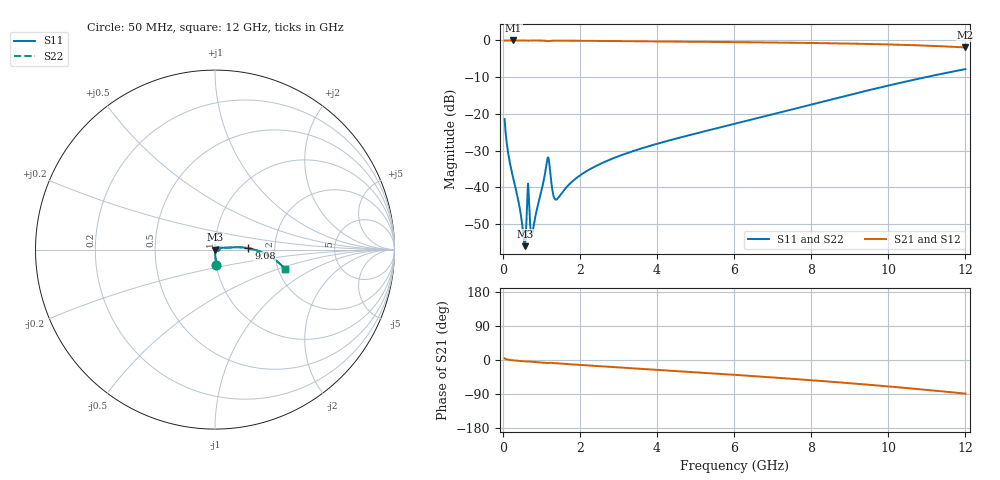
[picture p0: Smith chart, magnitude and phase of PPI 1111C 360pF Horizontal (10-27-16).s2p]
# MHz S MA R 50
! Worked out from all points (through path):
!   1601 points, 50 MHz to 12 GHz, reference 50 ohm
!   highest |S21| = 0.00 dB at 274.1 MHz (marker M1); lowest = -1.9 dB at 12 GHz (marker M2)
!   group delay of S21, straight-line fit = 20 ps
!   lowest |S11| = -56.0 dB at 572.8 MHz (marker M3), VSWR 1.00, Z = 50.2 - j0.0518 ohm
!   |S11| at or under -10 dB: start of sweep to 10.97 GHz
!   |S22| runs from -56.0 to -7.8 dB; largest |S21 - S12| = 0
!   S11 on the Smith chart (normalised r, x): 50 MHz: 1.00, -0.17; 9.08 GHz: 1.46, +0.02; 12 GHz: 2.19, -0.57
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50  0.08521 -84.6  0.9952 4.6  0.9952 4.6  0.08521 -84.6
162.0312  0.02546 -88.4  0.9992 0.4  0.9992 0.4  0.02546 -88.4
274.0625  0.0133 -89.0  0.9994 -0.9  0.9994 -0.9  0.0133 -89.0
423.4375  0.005922 -85.0  0.9992 -2.3  0.9992 -2.3  0.005922 -85.0
535.4688  0.002264 -60.7  0.9987 -3.2  0.9987 -3.2  0.002264 -60.7
572.8125  0.001588 -19.0  0.9984 -3.5  0.9984 -3.5  0.001588 -19.0
625.0938  0.004543 37.1  0.9965 -4.1  0.9965 -4.1  0.004543 37.1
662.4375  0.01078 -21.7  0.9897 -3.9  0.9897 -3.9  0.01078 -21.7
692.3125  0.0047 -48.0  0.9966 -4.1  0.9966 -4.1  0.0047 -48.0
752.0625  0.00229 -2.3  0.9977 -4.7  0.9977 -4.7  0.00229 -2.3
789.4062  0.002721 24.4  0.9976 -5.0  0.9976 -5.0  0.002721 24.4
1162.844  0.02481 20.5  0.978 -7.9  0.978 -7.9  0.02481 20.5
1215.125  0.02001 -21.1  0.9805 -7.3  0.9805 -7.3  0.02001 -21.1
1312.219  0.00791 -19.1  0.9922 -8.1  0.9922 -8.1  0.00791 -19.1
1379.438  0.006826 1.7  0.9932 -8.6  0.9932 -8.6  0.006826 1.7
2044.156  0.01506 31.2  0.9891 -13.3  0.9891 -13.3  0.01506 31.2
4038.312  0.03971 14.4  0.9692 -26.2  0.9692 -26.2  0.03971 14.4
6025  0.07355 8.4  0.9486 -39.2  0.9486 -39.2  0.07355 8.4
8019.156  0.1351 5.6  0.9235 -53.5  0.9235 -53.5  0.1351 5.6
9079.719  0.1861 2.4  0.9045 -61.9  0.9045 -61.9  0.1861 2.4
10013.31  0.244 -1.9  0.8818 -69.8  0.8818 -69.8  0.244 -1.9
12000  0.407 -15.5  0.8032 -88.8  0.8032 -88.8  0.407 -15.5
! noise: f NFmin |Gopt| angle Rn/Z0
50  0.0007391  0.9302  0.3242  0.002354
1372  0.009318  0.8548  8.522  0.01363
2701  0.02058  0.8712  16.67  0.03372
4031  0.03345  0.8837  24.63  0.05954
5360  0.04581  0.89  32.33  0.08364
6682  0.05761  0.8946  39.69  0.1056
8012  0.06938  0.8992  46.75  0.1269
9341  0.08158  0.9044  53.45  0.1494
1.067e+04  0.09481  0.9104  59.77  0.1751
1.2e+04  0.1098  0.9172  65.71  0.2066
